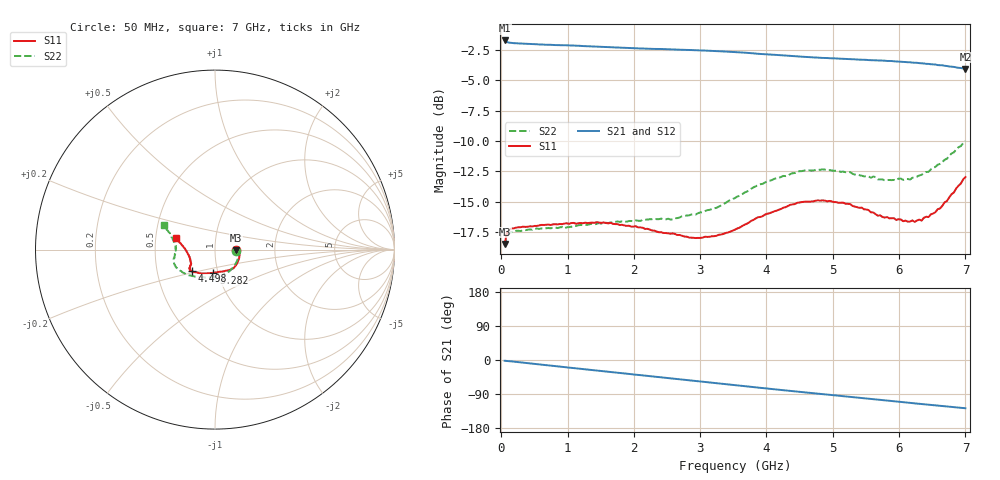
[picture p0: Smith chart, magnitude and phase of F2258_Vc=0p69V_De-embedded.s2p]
! Integrated Device Technology
! Corporate Headquarters
! 6024 Silver Creek Valley Road
! San Jose, CA 95138  USA
! Phone:  1-408-284-8200
! Toll Free:  1-800-223-1366
! Webpage:  http://www.idt.com/
! Timing and RF Division
! 515 Groton Road, Suite 102
! Westford, MA 01886-6024
! Device:  F2258
! Description: Voltage Variable RF Attenuator
! Frequency:  50.0 -  6000.00 MHz
! Package:  3x3 mm Thin QFN Plastic Package: 16 pin
! Ports:  2 RF, 2 DC
!  Pin  1  = NC
!  Pin  2  = NC
!  Pin  3  = RF2  = Port 2
!  Pin  4  = GND
!  Pin  5  = Vdd
!  Pin  6  = NC
!  Pin  7  = VCTRL
!  Pin  8  = NC
!  Pin  9  = GND
!  Pin 10  = RF1  = Port 1
!  Pin 11  = NC
!  Pin 12  = NC
!  Pin 13  = NC
!  Pin 14  = NC
!  Pin 15  = NC
!  Pin 16  = NC
! Vcntrl:  0.690 Volts
! Vdd:  +3.300 Volts
! Current:  1.121 mA
! Data:  The device was measured on a the F2258 evaluation board which has
!  individual transmission lines to the RF pins.  Data was collected
!  using a calibrated network analyzer.  The evaluation board was
!  de-embedded using a TRL calibration technique.
!  The reference plane is the edge of the package pin.
! Misc:  SN 10
!  Action Tracker AT0285
! Date Measured:  2014-12-10
! Date:  2016-01-13  MJV
! Note:
!  Integrated Device Technology supplies this data as a sample of measured
!  data at the package pin for this product.  Your particular data for this
!  product may vary.
!  Data was taken at 25 degrees C.
!  Integrated Device Technology reserves the right to change this data at anytime.
!Freq_(GHz)  S11M_(dB)  S11P_(deg)  S21M_(dB)  S21P_(deg)  S12M_(dB)  S12P_(deg)  S22M_(dB)  S22P_(deg)
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# GHz S dB R 50
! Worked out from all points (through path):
!   201 points, 50 MHz to 7 GHz, reference 50 ohm
!   highest |S21| = -1.71 dB at 50 MHz (marker M1); lowest = -4.1 dB at 7 GHz (marker M2)
!   group delay of S21, straight-line fit = 50.4 ps
!   lowest |S11| = -18.5 dB at 50 MHz (marker M3), VSWR 1.27, Z = 63.5 - j0.5 ohm
!   |S11| at or under -10 dB: start of sweep to end of sweep
!   |S22| runs from -18.7 to -10.0 dB; largest |S21 - S12| = 0.0016
!   S11 on the Smith chart (normalised r, x): 50 MHz: 1.27, -0.01; 3.282 GHz: 0.95, -0.25; 4.498 GHz: 0.75, -0.19; 7 GHz: 0.64, +0.08
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0.05  -18.49 -1.9  -1.71 -2.0  -1.71 -2.0  -18.67 -2.6
0.08475  -17.61 -3.2  -1.84 -2.5  -1.84 -2.5  -17.82 -4.0
0.15425  -17.22 -5.1  -1.92 -3.7  -1.91 -3.7  -17.50 -7.0
0.71025  -16.89 -22.7  -2.07 -14.2  -2.05 -14.2  -17.18 -29.4
0.9535  -16.81 -31.0  -2.11 -18.8  -2.10 -18.8  -17.21 -40.1
1.2315  -16.78 -38.1  -2.17 -24.0  -2.18 -24.0  -16.92 -50.0
1.6485  -16.75 -46.8  -2.28 -31.6  -2.27 -31.6  -16.71 -62.8
2.37825  -17.52 -61.3  -2.41 -44.8  -2.42 -44.8  -16.45 -82.6
2.58675  -17.62 -66.7  -2.45 -48.7  -2.45 -48.7  -16.46 -89.1
2.93425  -18.00 -78.7  -2.52 -55.1  -2.52 -55.1  -16.06 -101.5
3.28175  -17.73 -93.7  -2.60 -61.7  -2.60 -61.7  -15.41 -115.5
3.525  -17.31 -105.2  -2.68 -66.3  -2.68 -66.3  -14.70 -125.0
3.8725  -16.28 -119.5  -2.81 -72.8  -2.80 -72.8  -13.63 -137.6
4.498  -15.07 -136.6  -3.04 -84.1  -3.03 -84.1  -12.49 -154.8
4.7065  -14.98 -139.1  -3.11 -87.8  -3.10 -87.8  -12.44 -158.9
5.2625  -15.20 -144.9  -3.27 -97.3  -3.26 -97.3  -12.57 -168.0
5.85325  -16.38 -152.5  -3.41 -107.6  -3.40 -107.6  -13.22 -179.0
6.166  -16.65 -160.5  -3.51 -113.1  -3.51 -113.1  -13.18 174.3
6.2355  -16.67 -164.1  -3.55 -114.3  -3.54 -114.3  -12.99 172.2
6.444  -16.27 -173.1  -3.65 -118.0  -3.65 -118.0  -12.54 167.3
6.722  -14.95 173.7  -3.82 -122.9  -3.84 -122.9  -11.47 159.9
7  -12.97 163.7  -4.06 -127.3  -4.07 -127.3  -10.00 154.5
